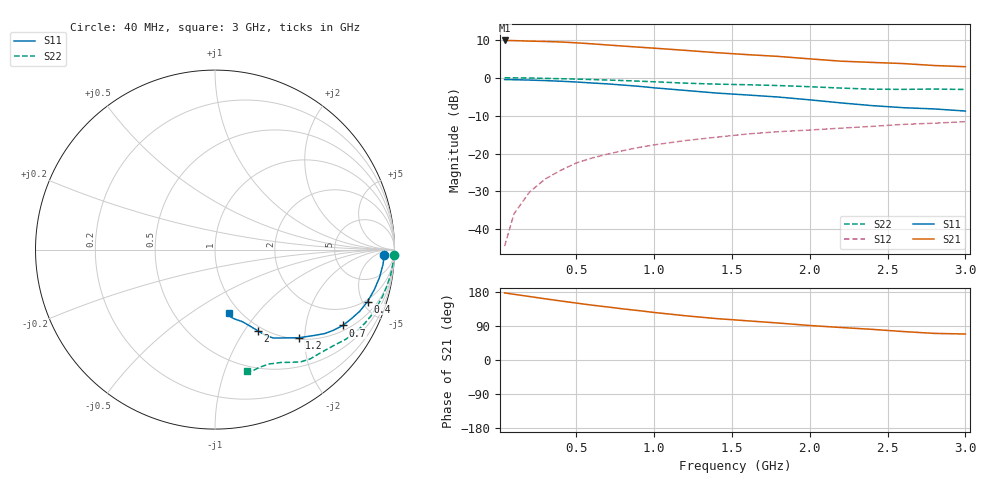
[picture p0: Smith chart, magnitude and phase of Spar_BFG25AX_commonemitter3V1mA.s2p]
! Filename:  BFG25AXI.S2P  Version:  2.0
! NXP part #: BFG25A/X  Date: May 1990
! Bias condition: Vce=3.0V, Ic=1.0mA
#  MHz  S  MA  R  50
! Freq  S11  S21  S12  S22  !GUM [dB]
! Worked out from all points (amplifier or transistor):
!   21 points, 40 MHz to 3 GHz, reference 50 ohm
!   highest |S21| = 9.8 dB at 40 MHz (marker M1)
!   |S21| within 3 dB of that: start of sweep to 1.329 GHz
!   unconditionally stable (mu >= 1): nowhere
!   at 300 MHz: K = 0.12, MSG = 18.1 dB, |S12| = -26.7 dB
!   at 1 GHz: K = 0.37, MSG = 12.8 dB, |S12| = -17.7 dB
!   at 3 GHz: K = 0.81, MSG = 7.2 dB, |S12| = -11.6 dB
!   lowest NFmin = 1.70 dB at 500 MHz
!   S11 on the Smith chart (normalised r, x): 40 MHz: 26, -15; 400 MHz: 1.82, -5.45; 700 MHz: 1.20, -3.23; 1.2 GHz: 1.03, -1.88; 2 GHz: 0.94, -1.15; 3 GHz: 0.89, -0.72
40  0.943 -1.9  3.095 177.1  0.006 89.8  0.998 -1.6
100  0.94 -4.9  3.08 173.4  0.016 87.7  0.995 -4.0
200  0.93 -9.5  3.034 167.5  0.031 83.4  0.989 -8.0
300  0.915 -14.2  3 161.5  0.046 80.4  0.979 -12.0
400  0.898 -18.8  2.956 155.8  0.06 77.3  0.969 -15.7
500  0.877 -23.0  2.882 150.3  0.075 74.6  0.957 -19.4
600  0.851 -27.0  2.795 144.8  0.087 72.6  0.945 -22.9
700  0.828 -30.7  2.7 140.0  0.098 70.4  0.931 -26.0
800  0.799 -34.2  2.611 134.9  0.109 68.5  0.916 -29.0
900  0.77 -37.4  2.527 130.4  0.12 66.5  0.9 -31.8
1000  0.735 -40.5  2.449 125.5  0.13 64.5  0.883 -34.5
1200  0.679 -46.3  2.292 116.8  0.148 60.3  0.847 -39.5
1400  0.627 -51.7  2.137 109.3  0.164 58.0  0.822 -44.5
1600  0.591 -56.5  2.012 103.4  0.181 55.9  0.807 -49.1
1800  0.555 -59.5  1.906 97.5  0.194 53.4  0.787 -52.6
2000  0.51 -62.3  1.77 91.0  0.204 51.3  0.76 -55.7
2200  0.465 -65.7  1.65 85.8  0.216 49.2  0.729 -59.6
2400  0.428 -69.4  1.589 80.9  0.228 46.9  0.705 -64.7
2600  0.402 -74.2  1.535 75.1  0.242 44.0  0.701 -69.4
2800  0.387 -76.7  1.446 70.2  0.251 42.8  0.707 -72.8
3000  0.363 -78.0  1.395 68.6  0.263 42.8  0.699 -75.4
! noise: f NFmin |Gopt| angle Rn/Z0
500  1.7  0.83  5  2.6
1000  1.8  0.78  13  2.8
2000  2.1  0.76  37  2
